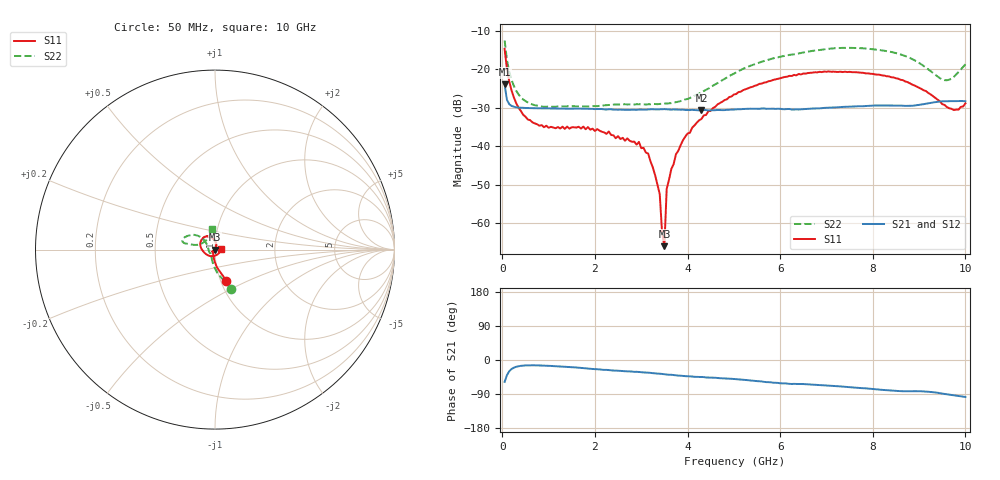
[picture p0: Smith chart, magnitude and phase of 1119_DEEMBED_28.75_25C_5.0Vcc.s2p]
!Hittite Microwave Corp.
!Digital Attenuator/PhaseShifter Rev 1.4.0
!Filename: C:\DATA\DATA\1119_DEEMBED_28.75_25C_5.0Vcc.s2p
!VNA ID: Agilent Technologies,N5224A,MY51441122,A.10.45.03
!Device type:
!2 Port Calibration.
!Temp(C): 25
!Lot Number:
!Serial Number:
!Operator:
!Misc:
!Attenuator:  28.750
# GHZ S DB R 50.0
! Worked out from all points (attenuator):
!   200 points, 50 MHz to 10 GHz, reference 50 ohm
!   highest |S21| = -23.99 dB at 50 MHz (marker M1); lowest = -30.7 dB at 4.3 GHz (marker M2)
!   lowest |S11| = -66.0 dB at 3.5 GHz (marker M3), VSWR 1.00, Z = 50 + j0.0299 ohm
!   |S11| at or under -10 dB: start of sweep to end of sweep
!   |S22| runs from -29.8 to -12.6 dB; largest |S21 - S12| = 0.00012
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0.05  -14.74 -70.0  -23.99 -57.8  -23.99 -57.8  -12.56 -67.5
0.1  -19.96 -83.5  -27.98 -40.0  -27.98 -39.9  -17.51 -84.0
0.2  -25.55 -96.0  -29.56 -23.8  -29.56 -23.8  -22.78 -100.6
0.35  -30.00 -107.3  -29.99 -16.5  -29.98 -16.5  -26.56 -114.7
0.55  -33.08 -120.1  -30.11 -14.1  -30.11 -14.1  -28.66 -126.5
0.9  -35.10 -131.9  -30.19 -14.8  -30.20 -14.8  -29.77 -135.9
1.75  -34.93 -138.8  -30.29 -21.4  -30.29 -21.5  -29.67 -140.9
2.95  -38.91 -112.5  -30.50 -31.6  -30.51 -31.6  -29.14 -160.2
3.15  -41.93 -103.7  -30.48 -33.4  -30.50 -33.4  -29.13 -166.2
3.4  -52.47 -109.0  -30.45 -36.2  -30.46 -36.3  -29.05 -173.7
3.45  -62.39 -48.0  -30.44 -36.9  -30.45 -37.0  -28.98 -175.6
3.5  -65.98 36.4  -30.39 -37.4  -30.40 -37.5  -28.93 -177.3
3.55  -51.11 67.1  -30.43 -38.5  -30.44 -38.5  -28.93 -179.2
3.65  -45.94 56.9  -30.52 -39.0  -30.52 -39.1  -28.82 177.1
3.9  -38.51 67.3  -30.53 -42.1  -30.55 -42.1  -28.09 166.4
4.3  -32.94 73.7  -30.72 -44.7  -30.73 -44.8  -25.99 150.4
5.05  -26.47 89.4  -30.46 -50.5  -30.48 -50.6  -20.83 138.6
6.7  -20.91 127.4  -30.24 -65.0  -30.25 -65.0  -15.26 153.8
8.35  -21.90 170.8  -29.46 -80.0  -29.46 -80.1  -15.44 168.1
9.55  -29.31 -90.3  -28.34 -89.6  -28.36 -89.7  -22.87 138.1
9.85  -30.55 -25.8  -28.29 -94.8  -28.30 -94.8  -20.77 105.8
10  -28.90 2.8  -28.34 -97.6  -28.34 -97.5  -18.74 98.2
